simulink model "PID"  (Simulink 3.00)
settings: Solver=ode45  StartTime=0.0  StopTime=40  RelTol=1e-3
libraries: simulink3 x1

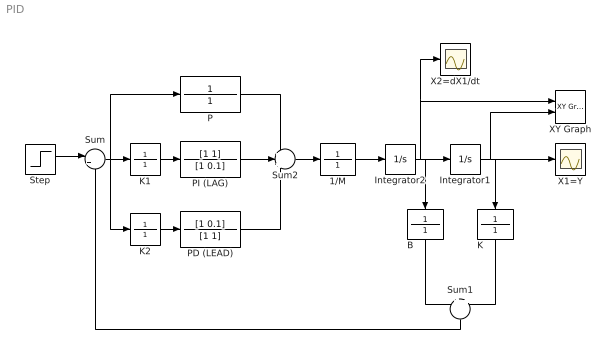
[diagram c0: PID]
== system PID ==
  1/M : TransferFcn  Numerator=1  Denominator=1
  B : TransferFcn  Orientation=down  Numerator=1  Denominator=1
  Integrator1 : Integrator  ExternalReset=none  InitialConditionSource=internal  InitialCondition=0  LimitOutput=off  UpperSaturationLimit=inf  LowerSaturationLimit=-inf  ShowSaturationPort=off  ShowStatePort=off  AbsoluteTolerance=auto
  Integrator2 : Integrator  ExternalReset=none  InitialConditionSource=internal  InitialCondition=0  LimitOutput=off  UpperSaturationLimit=inf  LowerSaturationLimit=-inf  ShowSaturationPort=off  ShowStatePort=off  AbsoluteTolerance=auto
  K : TransferFcn  Orientation=down  Numerator=1  Denominator=1
  K1 : TransferFcn  Numerator=1  Denominator=1
  K2 : TransferFcn  Numerator=1  Denominator=1
  P : TransferFcn  Numerator=1  Denominator=1
  PD (LEAD) : TransferFcn  Numerator=[1 0.1]  Denominator=[1 1]
  PI (LAG) : TransferFcn  Numerator=[1 1]  Denominator=[1 0.1]
  Step : Step  Time=0  Before=0  After=1  SampleTime=0
  Sum : Sum  Inputs=|+-  SaturateOnIntegerOverflow=on
  Sum1 : Sum  Orientation=down  Inputs=+||+  SaturateOnIntegerOverflow=on
  Sum2 : Sum  Inputs=+++  SaturateOnIntegerOverflow=on
  X1=Y : Scope
  X2=dX1/dt : Scope
  XY Graph : simulink3/Sinks/XY Graph  xmin=-1  xmax=2  ymin=-1  ymax=1  st=.1
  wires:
  Step/1 -> Sum/1
  Sum1/1 -> Sum/2
  Integrator1/1 -> X1=Y/1, K/1, XY Graph/2
  1/M/1 -> Integrator2/1
  Integrator2/1 -> Integrator1/1, B/1, X2=dX1/dt/1, XY Graph/1
  Sum/1 -> P/1, K1/1, K2/1
  K1/1 -> PI (LAG)/1
  K2/1 -> PD (LEAD)/1
  K/1 -> Sum1/2
  B/1 -> Sum1/1
  Sum2/1 -> 1/M/1
  PI (LAG)/1 -> Sum2/2
  P/1 -> Sum2/1
  PD (LEAD)/1 -> Sum2/3
